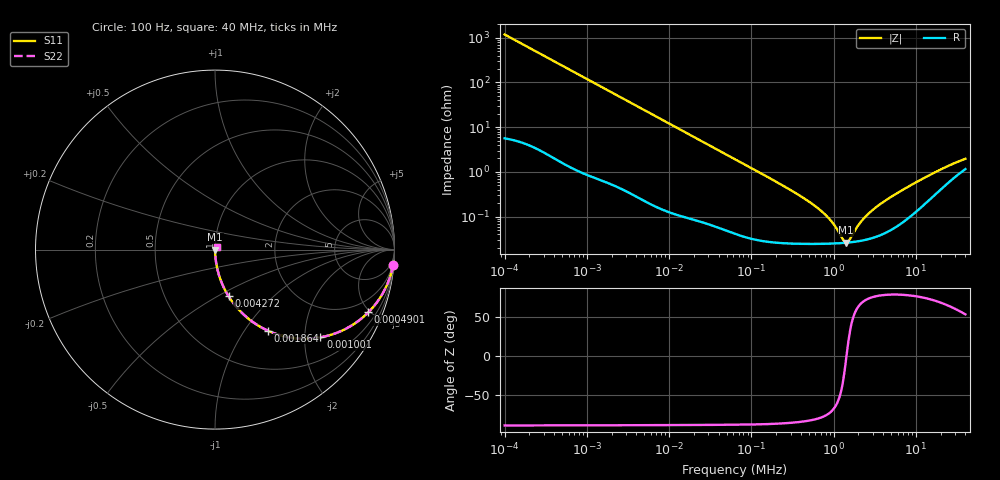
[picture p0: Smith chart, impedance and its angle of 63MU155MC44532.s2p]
!Components F PML CAP
!CONCATENATE F 0.1-40000kHz, at 20deg DC=0V
!Part Number F 63MU155MC44532
!Copyright(C) Rubycon Corporation. 20160805
# MHz S MA R 50
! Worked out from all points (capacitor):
!   561 points, 100 Hz to 40 MHz, reference 50 ohm
!   read as one part in series: C = 1.34 uF near 104.7 Hz
!   lowest |Z| = 26.3 mohm at 1.418 MHz (marker M1)
!   series resonance near 1.434 MHz, so ESL is about 9.2 nH
!   S11 on the Smith chart (normalised r, x): 100 Hz: 1, -24; 490.1 Hz: 1.03, -4.87; 1.001 kHz: 1.02, -2.39; 1.864 kHz: 1.01, -1.29; 4.272 kHz: 1.01, -0.56; 40 MHz: 1.02, +0.03
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0.0001  0.9961 -4.8  0.08412 84.9  0.08412 84.9  0.9961 -4.8
0.0002571289  0.9761 -12.2  0.211 77.4  0.211 77.4  0.9761 -12.2
0.0004900652  0.9229 -22.3  0.379 67.3  0.379 67.3  0.9229 -22.3
0.0008716573  0.8054 -36.0  0.5872 53.6  0.5872 53.6  0.8054 -36.0
0.001000847  0.7642 -39.8  0.6395 49.8  0.6395 49.8  0.7642 -39.8
0.001864091  0.5391 -56.9  0.8376 32.6  0.8376 32.6  0.5391 -56.9
0.00275759  0.3985 -66.0  0.9135 23.5  0.9135 23.5  0.3985 -66.0
0.004271689  0.2711 -73.7  0.96 15.7  0.96 15.7  0.2711 -73.7
0.007424854  0.1605 -80.2  0.9855 9.2  0.9855 9.2  0.1605 -80.2
0.01823188  0.0664 -85.4  0.9969 3.8  0.9969 3.8  0.0664 -85.4
0.06324555  0.01937 -87.7  0.9994 1.1  0.9994 1.1  0.01937 -87.7
0.2637898  0.004523 -86.5  0.9997 0.3  0.9997 0.3  0.004523 -86.5
0.5512845  0.001922 -82.5  0.9998 0.1  0.9998 0.1  0.001922 -82.5
0.8942378  0.0008786 -73.4  0.9998 0.0  0.9998 0.0  0.0008786 -73.4
1.322865  0.0002938 -28.1  0.9997 0.0  0.9997 0.0  0.0002938 -28.1
1.417512  0.0002625 -4.2  0.9997 0.0  0.9997 0.0  0.0002625 -4.2
1.554323  0.0003003 27.6  0.9997 -0.0  0.9997 -0.0  0.0003003 27.6
1.956943  0.0006118 62.6  0.9997 -0.0  0.9997 -0.0  0.0006118 62.6
2.463854  0.001023 72.6  0.9997 -0.1  0.9997 -0.1  0.001023 72.6
4.69589  0.002581 79.3  0.9995 -0.1  0.9995 -0.1  0.002581 79.3
15.5564  0.008973 72.4  0.9973 -0.5  0.9973 -0.5  0.008973 72.4
40  0.01947 53.1  0.9884 -0.9  0.9884 -0.9  0.01947 53.1
